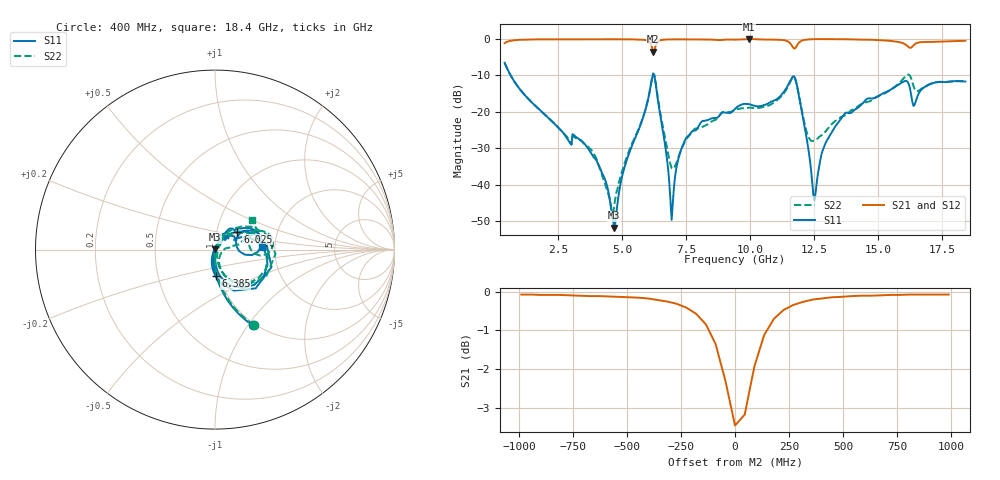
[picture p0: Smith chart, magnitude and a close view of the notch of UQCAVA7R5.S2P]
!  Part Number  UQCAVA7R5	Mounting Orientation: Horizontal
!  Description: RF capacitors
!  Application: Coupling, Bypass, Tuning, DC Block
!  Filters, Matching
# GHZ S DB R 50
! Freq  |S11|  S11 Ph  |S21|  S21 Ph  |S12|  S12 Ph  |S22|  S22 Ph
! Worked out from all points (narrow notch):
!   401 points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, 400 MHz to 18.4 GHz, reference 50 ohm
!   highest |S21| = 0.00 dB at 9.94 GHz (marker M1); lowest = -3.5 dB at 6.205 GHz (marker M2)
!   notch at M2: 3.3 dB deep, 166 MHz wide at half that depth
!   lowest |S11| = -51.8 dB at 4.675 GHz (marker M3), VSWR 1.01, Z = 49.9 + j0.242 ohm
!   |S11| at or under -10 dB: 638.7 MHz to 6.191 GHz (5.552 GHz wide, 163 % of centre); 6.241 GHz to end of sweep
!   |S22| runs from -49.2 to -6.5 dB; largest |S21 - S12| = 0.0024
!   S11 on the Smith chart (normalised r, x): 400 MHz: 0.97, -1.06; 6.025 GHz: 1.26, +0.26; 6.385 GHz: 0.96, -0.29; 18.4 GHz: 1.70, +0.06
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0.4  -6.51 -63.4  -1.11 26.7  -1.11 26.7  -6.51 -62.8
3.415  -28.03 -103.7  -0.05 -10.4  -0.05 -10.4  -28.11 -91.0
4.27  -37.68 -114.3  -0.05 -14.8  -0.06 -14.8  -38.84 -90.4
4.675  -51.82 109.2  -0.04 -16.9  -0.04 -16.9  -45.97 17.4
5.08  -35.33 72.3  -0.06 -19.2  -0.06 -19.2  -34.25 54.7
6.025  -15.91 38.5  -0.57 -29.9  -0.57 -29.9  -15.79 46.9
6.205  -9.64 -17.2  -3.46 -26.9  -3.46 -26.9  -9.41 -4.0
6.385  -16.60 -88.8  -0.70 -14.0  -0.70 -14.0  -16.13 -69.3
6.43  -18.72 -95.3  -0.47 -15.7  -0.47 -15.6  -18.14 -73.7
6.925  -49.65 155.0  -0.08 -23.2  -0.08 -23.2  -35.43 -30.4
7.51  -27.01 56.9  -0.07 -27.1  -0.07 -27.0  -27.34 44.8
9.4  -19.17 43.4  -0.15 -35.7  -0.15 -35.6  -19.47 53.1
9.94  -17.86 28.0  0.00 -38.2  -0.01 -38.2  -18.84 47.7
11.695  -10.21 -28.2  -2.54 -47.4  -2.54 -47.4  -10.39 -20.7
12.415  -39.15 -64.3  -0.03 -44.6  -0.03 -44.6  -28.05 -32.0
12.55  -42.08 30.9  -0.01 -45.8  -0.01 -45.8  -27.67 -18.9
12.865  -29.83 69.2  -0.01 -48.0  -0.01 -48.0  -25.99 0.2
13.63  -21.07 67.1  -0.03 -52.8  -0.03 -52.8  -21.13 7.6
15.43  -14.05 37.3  -0.48 -63.5  -0.47 -63.5  -14.18 21.8
16.105  -11.53 8.8  -1.72 -68.2  -1.71 -68.2  -9.94 13.8
16.42  -17.97 22.0  -1.42 -57.7  -1.41 -57.8  -13.78 -2.1
18.4  -11.65 3.6  -0.46 -71.3  -0.46 -71.4  -11.56 38.0
